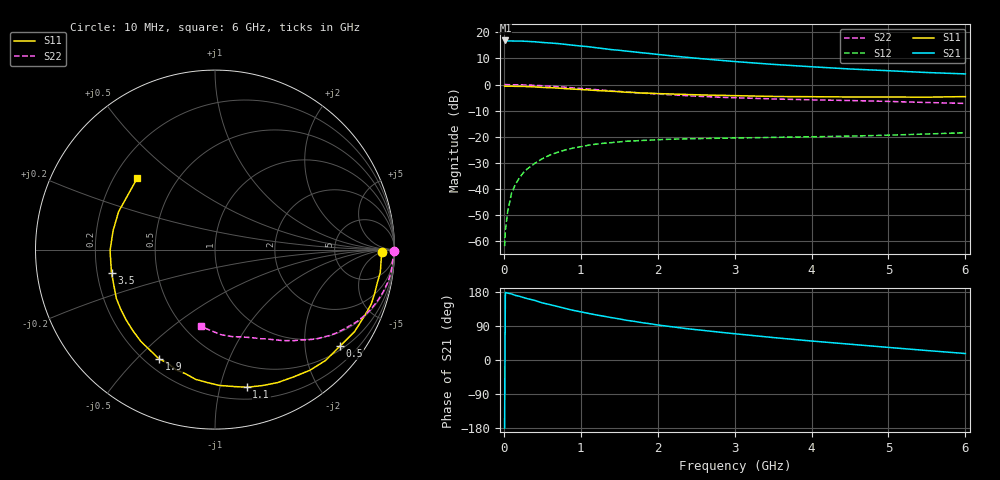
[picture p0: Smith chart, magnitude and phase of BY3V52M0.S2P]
! SIEMENS Small Signal Semiconductors
! BFY420
! Si NPN RF SIEGET Grounded Emitter Transistor in MICRO-X
! VCE = 3.5 V  IC = 2 mA
! Common Emitter S-Parameters:  October  1996
# GHz  S  MA  R  50
!  f  S11  S21  S12  S22
! GHz  MAG  ANG  MAG  ANG  MAG  ANG  MAG  ANG
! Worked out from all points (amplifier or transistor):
!   36 points, 10 MHz to 6 GHz, reference 50 ohm
!   highest |S21| = 16.9 dB at 20 MHz (marker M1)
!   |S21| within 3 dB of that: start of sweep to 1.262 GHz
!   unconditionally stable (mu >= 1): 4.027 GHz to end of sweep
!   at 250 MHz: K = 0.06, MSG = 25.3 dB, |S12| = -33.9 dB
!   at 1.4 GHz: K = 0.28, MSG = 17.8 dB, |S12| = -22.2 dB
!   at 6 GHz: K = 1.23, MAG = 8.4 dB, |S12| = -18.5 dB
!   S11 on the Smith chart (normalised r, x): 10 MHz: 27, -6; 500 MHz: 0.59, -2.81; 1.1 GHz: 0.30, -1.21; 1.9 GHz: 0.25, -0.58; 3.5 GHz: 0.26, -0.10; 6 GHz: 0.30, +0.36
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0.01  0.9307 -0.9  6.985 -179.7  0.0008 86.9  0.9972 -0.4
0.02  0.9284 -1.5  6.994 178.4  0.0016 74.1  0.998 -0.7
0.05  0.9275 -3.9  6.861 176.4  0.0037 87.0  0.995 -1.8
0.1  0.9297 -7.8  6.837 174.4  0.0083 86.5  0.9916 -3.6
0.15  0.9229 -11.6  6.814 170.4  0.0122 81.6  0.9902 -5.5
0.25  0.9218 -19.1  6.782 165.2  0.0201 78.0  0.9842 -9.0
0.4  0.9021 -30.5  6.601 157.3  0.0307 72.3  0.9655 -14.3
0.5  0.8797 -37.8  6.401 150.8  0.0379 68.7  0.9484 -17.7
0.7  0.8554 -51.8  6.099 141.1  0.0503 61.0  0.91 -23.9
0.8  0.8331 -58.5  5.887 136.0  0.0559 56.8  0.8872 -26.9
0.9  0.8188 -64.8  5.671 131.1  0.0606 54.0  0.8635 -29.4
1.1  0.7873 -77.0  5.303 123.0  0.0688 48.3  0.8201 -34.5
1.4  0.7421 -93.2  4.665 111.8  0.0772 40.9  0.7594 -40.7
1.6  0.71 -103.7  4.36 104.6  0.0821 36.6  0.7185 -44.4
1.9  0.6841 -117.2  3.927 95.7  0.086 31.7  0.6712 -49.1
2.2  0.6579 -128.7  3.52 87.3  0.0899 27.7  0.6334 -53.2
2.4  0.6429 -135.4  3.298 82.2  0.0913 25.8  0.6088 -55.8
2.8  0.6212 -147.9  2.922 73.5  0.0937 22.7  0.5714 -60.4
3.5  0.591 -167.3  2.436 59.3  0.0972 19.3  0.5299 -67.7
4.5  0.5775 169.4  1.986 41.7  0.1028 16.9  0.4938 -79.0
5.5  0.5729 147.6  1.7 25.0  0.1128 16.2  0.4528 -92.6
6  0.5879 137.6  1.598 17.1  0.1193 15.5  0.4347 -100.5
